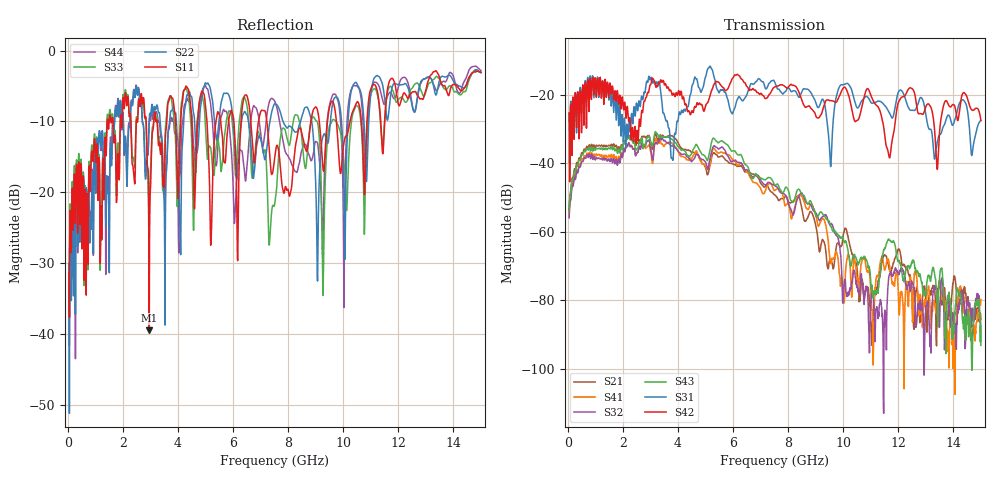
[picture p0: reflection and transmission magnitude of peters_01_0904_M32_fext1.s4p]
# MHZ S RI R 50.00
! FREQ  S11  S12  S13  S14
!  S21  S22  S23  S24
!  S31  S32  S33  S34
!  S41  S42  S43  S44
!  REAL  IMAG  REAL  IMAG  REAL  IMAG  REAL  IMAG
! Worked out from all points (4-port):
!   1496 points, 50 MHz to 15 GHz, reference 50 ohm
!   strongest paths, dB at 50 MHz, 3.79 GHz, 7.53 GHz, 11.27 GHz, 15 GHz:
!     S42: -25.4, -20.0, -17.6, -23.5, -27.5
!     S31: -25.4, -38.5, -16.6, -21.8, -27.4
!     S43: -54.0, -33.0, -46.4, -78.0, -93.2
!     S32: -55.9, -34.9, -46.6, -85.4, -89.5
!     S41: -55.4, -34.2, -47.9, -72.8, -79.8
!     S21: -53.6, -31.9, -49.3, -74.4, -85.6
!   lowest |S11| = -39.4 dB at 2.96 GHz (marker M1), VSWR 1.02, Z = 50 - j1.07 ohm
!   |S11| at or under -10 dB: start of sweep to 1.432 GHz; 7.229 GHz to 8.827 GHz (1.598 GHz wide, 19.9 % of centre); 9.754 GHz to 10.25 GHz (493.9 MHz wide, 4.94 % of centre)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
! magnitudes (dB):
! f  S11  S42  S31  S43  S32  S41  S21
! 50 MHz  -31.3  -25.4  -25.4  -54.0  -55.9  -55.4  -53.6
! 2.96 GHz  -39.4  -18.2  -14.8  -32.1  -33.3  -34.7  -32.0
! 3.79 GHz  -6.7  -20.0  -38.5  -33.0  -34.9  -34.2  -31.9
! 5.15 GHz  -19.2  -20.7  -11.7  -36.8  -39.2  -40.8  -41.2
! 9.07 GHz  -8.5  -26.7  -23.6  -55.8  -55.5  -57.7  -61.2
! 10.17 GHz  -11.5  -19.5  -16.7  -65.2  -78.8  -66.6  -61.1
! 15 GHz  -3.1  -27.5  -27.4  -93.2  -89.5  -79.8  -85.6
